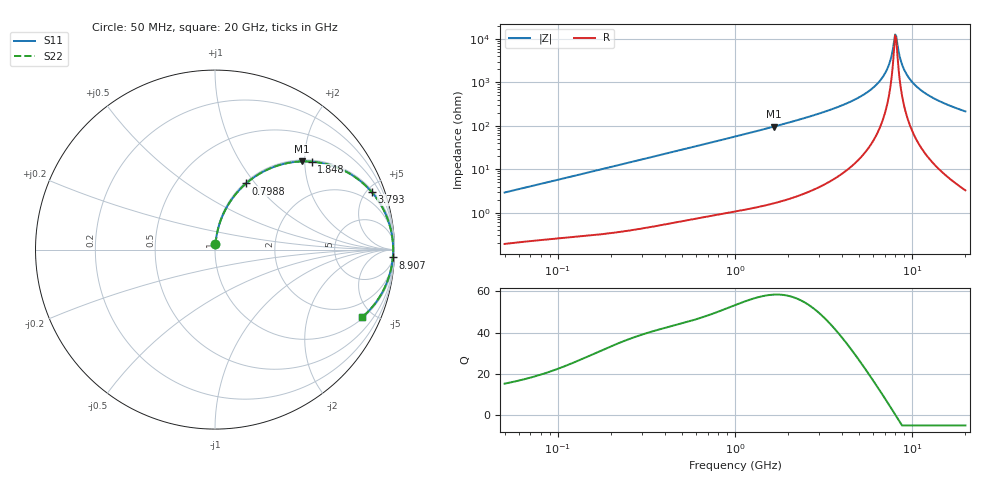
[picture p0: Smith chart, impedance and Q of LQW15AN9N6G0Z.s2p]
!Murata Part Number: LQW15AN9N6G0Z
!These Parameters are Measured in Series Mode Connection
!  o--[Z]--o
!Port1  Port2
!  o-------o
!Freq. Start=50[MHz] Stop=20[GHz], 401[Steps]
# Hz S RI R 50
!Freq.(Hz) S11(Real) S11(Imag) S21(Real) S21(Imag) S12(Real) S12(Imag) S22(Real) S22(Imag)
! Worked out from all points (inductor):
!   401 points, 50 MHz to 20 GHz, reference 50 ohm
!   read as one part in series: L = 9.2 nH near 51.52 MHz
!   highest Q = 58.4 at 1.664 GHz (marker M1), where L = 9.23 nH
!   self-resonance near 8.021 GHz
!   S11 on the Smith chart (normalised r, x): 50 MHz: 1.00, +0.06; 798.8 MHz: 1.02, +0.90; 1.848 GHz: 1.04, +2.16; 3.793 GHz: 1.13, +5.39; 8.907 GHz: 8, -44; 20 GHz: 1.07, -4.30
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5e7  0.00275 0.029  0.9973 -0.029  0.9973 -0.029  0.00275 0.029
1.364002e8  0.0088 0.0768  0.9912 -0.0768  0.9912 -0.0768  0.0088 0.0768
3.721004e8  0.0467 0.1992  0.9533 -0.1992  0.9533 -0.1992  0.0467 0.1992
7.987718e8  0.1735 0.3688  0.8265 -0.3688  0.8265 -0.3688  0.1735 0.3688
1e9  0.2465 0.4217  0.7535 -0.4217  0.7535 -0.4217  0.2465 0.4217
1.664083e9  0.4824 0.4912  0.5176 -0.4912  0.5176 -0.4912  0.4824 0.4912
1.848039e9  0.5388 0.49  0.4612 -0.49  0.4612 -0.49  0.5388 0.49
2.728004e9  0.7406 0.4289  0.2594 -0.4289  0.2594 -0.4289  0.7406 0.4289
3.792786e9  0.8731 0.3206  0.1269 -0.3206  0.1269 -0.3206  0.8731 0.3206
4.89267e9  0.9414 0.2177  0.0586 -0.2177  0.0586 -0.2177  0.9414 0.2177
5.944466e9  0.9737 0.134  0.0263 -0.134  0.0263 -0.134  0.9737 0.134
6.802353e9  0.9867 0.0749  0.0133 -0.0749  0.0133 -0.0749  0.9867 0.0749
7.442007e9  0.9912 0.0354  0.00878 -0.0354  0.00878 -0.0354  0.9912 0.0354
7.901521e9  0.9925 0.00896  0.00754 -0.00896  0.00754 -0.00896  0.9925 0.00896
8.020766e9  0.9926 0.00235  0.00745 -0.00235  0.00745 -0.00235  0.9926 0.00235
8.264682e9  0.9925 -0.0109  0.00753 0.0109  0.00753 0.0109  0.9925 -0.0109
8.644534e9  0.9917 -0.0307  0.00832 0.0307  0.00832 0.0307  0.9917 -0.0307
8.907419e9  0.9907 -0.0439  0.00929 0.0439  0.00929 0.0439  0.9907 -0.0439
9.892087e9  0.9845 -0.0901  0.0155 0.0901  0.0155 0.0901  0.9845 -0.0901
1.166392e10  0.9656 -0.1621  0.0344 0.1621  0.0344 0.1621  0.9656 -0.1621
1.482269e10  0.917 -0.2639  0.083 0.2639  0.083 0.2639  0.917 -0.2639
2e10  0.8184 -0.378  0.1816 0.378  0.1816 0.378  0.8184 -0.378
